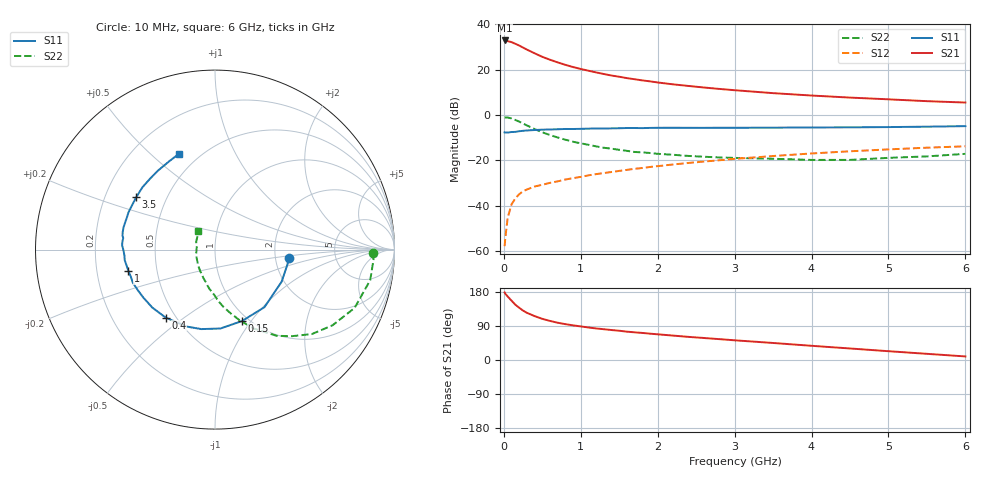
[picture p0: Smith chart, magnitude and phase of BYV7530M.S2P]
! SIEMENS Small Signal Semiconductors
! BFY420
! Si NPN RF SIEGET Grounded Emitter Transistor in MICRO-X
! VCE = 0.75 V  IC = 30 mA
! Common Emitter S-Parameters:  October  1996
# GHz  S  MA  R  50
!  f  S11  S21  S12  S22
! GHz  MAG  ANG  MAG  ANG  MAG  ANG  MAG  ANG
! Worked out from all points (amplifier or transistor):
!   36 points, 10 MHz to 6 GHz, reference 50 ohm
!   highest |S21| = 32.8 dB at 10 MHz (marker M1)
!   |S21| within 3 dB of that: start of sweep to 241.9 MHz
!   unconditionally stable (mu >= 1): start of sweep to 19.76 MHz; 1.273 GHz to end of sweep
!   at 250 MHz: K = 0.41, MSG = 31.6 dB, |S12| = -33.6 dB
!   at 1.4 GHz: K = 1.03, MAG = 20.1 dB, |S12| = -25.1 dB
!   at 6 GHz: K = 1.12, MAG = 7.6 dB, |S12| = -13.8 dB
!   S11 on the Smith chart (normalised r, x): 10 MHz: 2.39, -0.25; 150 MHz: 0.93, -0.90; 400 MHz: 0.44, -0.43; 1 GHz: 0.34, -0.11; 3.5 GHz: 0.33, +0.27; 6 GHz: 0.39, +0.62
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0.01  0.4151 -6.1  43.77 178.3  0.0013 97.1  0.8791 -1.2
0.02  0.412 -11.5  43.51 174.6  0.002 94.5  0.8847 -3.7
0.05  0.4121 -25.8  42.27 167.5  0.0055 84.4  0.8815 -11.1
0.1  0.4229 -49.4  40.27 156.6  0.0108 73.5  0.8429 -22.7
0.15  0.4255 -69.3  36.9 145.8  0.0147 68.0  0.7788 -32.8
0.2  0.4407 -86.1  33.84 137.8  0.0181 63.6  0.7159 -41.1
0.25  0.4493 -99.7  30.46 130.3  0.021 59.7  0.6459 -48.3
0.3  0.457 -110.2  27.53 124.5  0.023 57.6  0.5909 -54.4
0.4  0.4679 -126.0  22.83 115.8  0.0267 54.2  0.4909 -63.7
0.5  0.4758 -137.3  19.1 108.6  0.0292 53.9  0.4168 -70.8
0.6  0.4808 -146.5  16.46 103.1  0.0322 54.1  0.363 -76.5
0.7  0.4864 -152.8  14.4 98.3  0.0347 54.2  0.3207 -81.9
0.8  0.4936 -158.2  12.71 94.6  0.0381 54.3  0.2866 -86.4
1  0.4967 -166.0  10.31 88.6  0.0435 55.0  0.2383 -93.7
1.1  0.5013 -170.4  9.445 85.8  0.047 55.7  0.2211 -98.1
1.4  0.5083 -178.5  7.397 79.1  0.0558 55.9  0.1816 -108.3
1.6  0.5181 177.4  6.485 74.8  0.0621 55.5  0.1627 -115.5
2.2  0.5245 166.4  4.734 64.4  0.0817 53.3  0.1335 -132.6
3.5  0.5271 146.4  3.031 44.9  0.1252 44.5  0.109 -165.0
4.5  0.5357 132.6  2.42 30.4  0.1592 34.8  0.103 170.8
5.5  0.5541 117.5  2.018 16.3  0.191 24.4  0.1229 142.7
6  0.5697 110.8  1.883 9.4  0.205 19.1  0.1399 132.1
